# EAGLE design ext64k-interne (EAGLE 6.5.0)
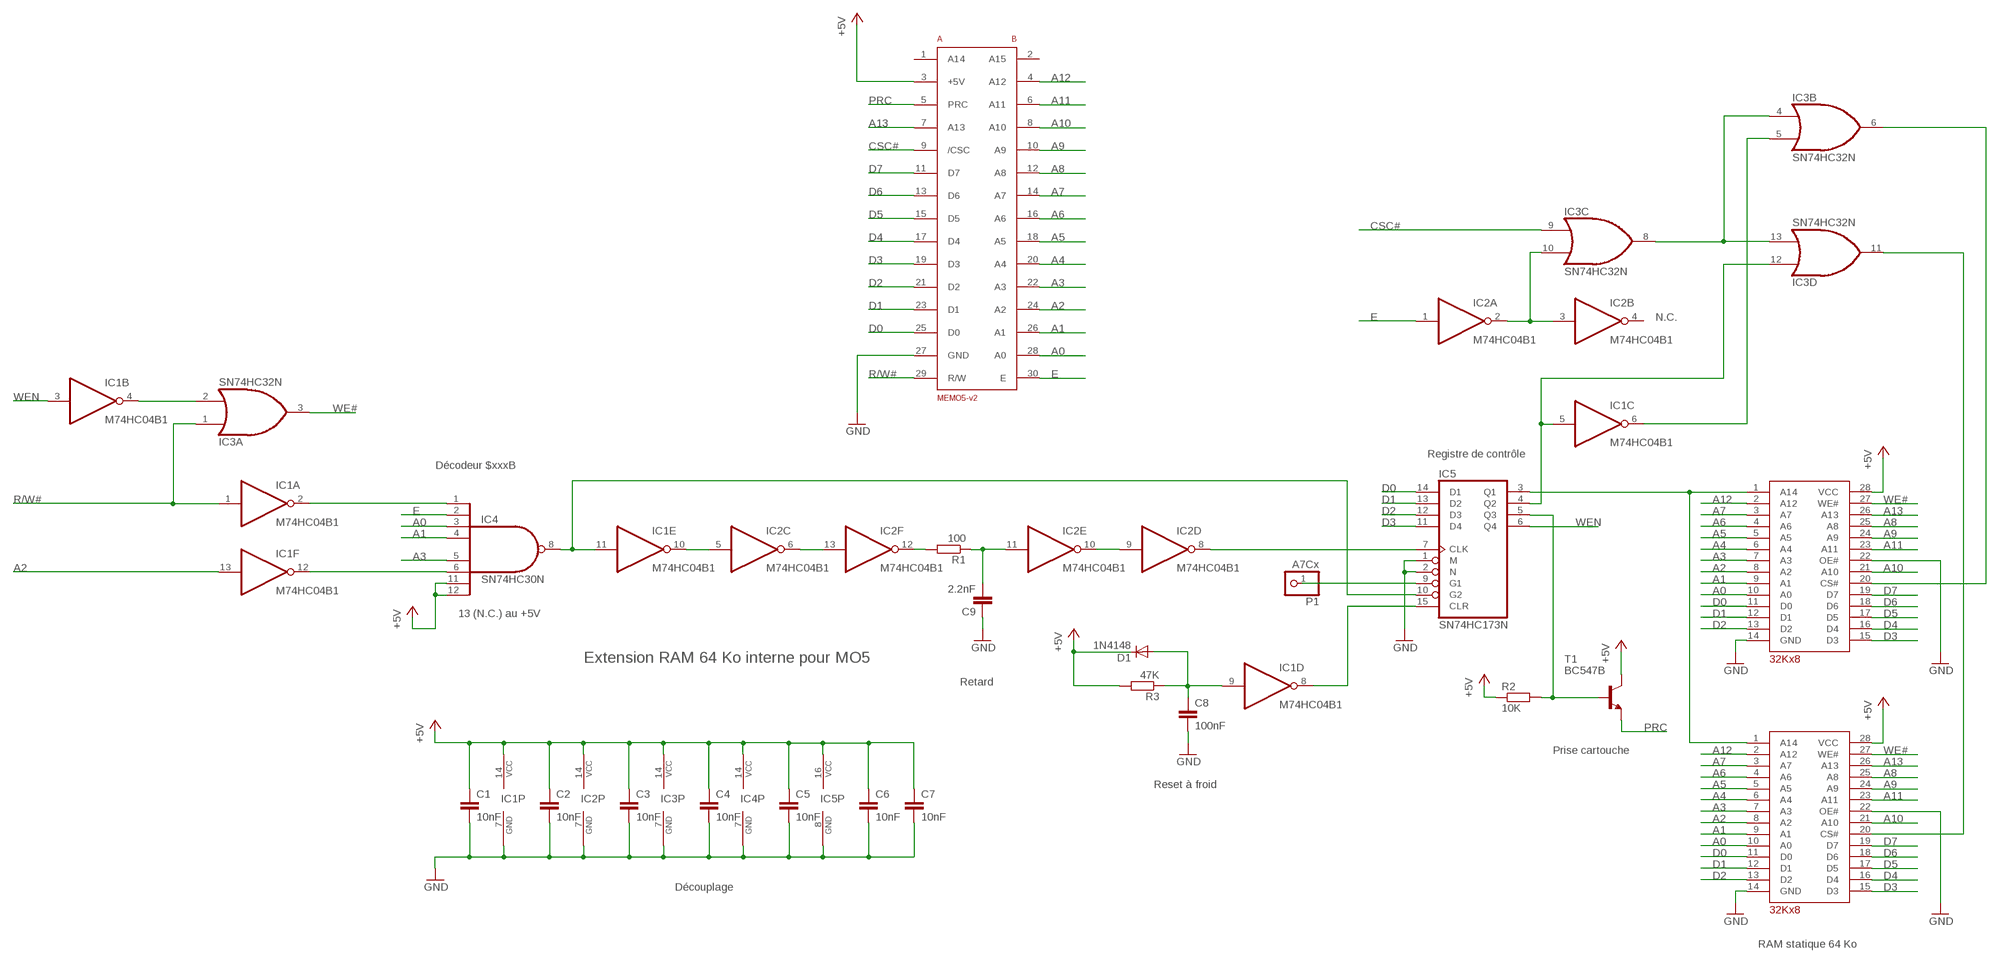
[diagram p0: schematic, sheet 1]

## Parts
C1  10nF  C-EU025-024X044  [C025-024X044]
C2  10nF  C-EU025-024X044  [C025-024X044]
C3  10nF  C-EU025-024X044  [C025-024X044]
C4  10nF  C-EU025-024X044  [C025-024X044]
C5  10nF  C-EU025-024X044  [C025-024X044]
C6  10nF  C-EU025-024X044  [C025-024X044]
C7  10nF  C-EU025-024X044  [C025-024X044]
C8  100nF  C-EU050-025X075  [C050-025X075]
C9  2.2nF  C-EU025-024X044  [C025-024X044]
D1  1N4148  1N4148DO35-10  [DO35-10]
IC1  M74HC04B1  74AS04N  [DIL14]
IC2  M74HC04B1  74AS04N  [DIL14]
IC3  SN74HC32N  74LS32N  [DIL14]
IC4  SN74HC30N  74ALS30N  [DIL14]
IC5  SN74HC173N  74LS173N  [DIL16]
IC6  D43256AC-10NL  D43256  [DIL28-6]
IC7  D43256AC-10NL  D43256  [DIL28-6]
P1  A7Cx  PINHD-1X1  [1X01]
R1  100  R-EU_0207/10  [0207/10]
R2  10K  R-EU_0207/10  [0207/10]
R3  47K  R-EU_0207/10  [0207/10]
T1  BC547B  BC547  [TO92]
U$1  MEMO5-V2HE  [HE15]

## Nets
+5V: C1.1 C2.1 C3.1 C4.1 C5.1 C6.1 C7.1 D1.C IC1.14(P:VCC) IC2.14(P:VCC) IC3.14(P:VCC) IC4.11(I6) IC4.12(I7) IC4.14(VCC) IC5.16(VCC) IC6.28(VCC) IC7.28(VCC) R2.1 R3.2 T1.3(C) U$1.3(+5V)
A0: IC4.3(I2) IC6.10(A0) IC7.10(A0) U$1.28(A0)
A1: IC4.4(I3) IC6.9(A1) IC7.9(A1) U$1.26(A1)
A2: IC1.13(F:I) IC6.8(A2) IC7.8(A2) U$1.24(A2)
A3: IC4.5(I4) IC6.7(A3) IC7.7(A3) U$1.22(A3)
A4: IC6.6(A4) IC7.6(A4) U$1.20(A4)
A5: IC6.5(A5) IC7.5(A5) U$1.18(A5)
A6: IC6.4(A6) IC7.4(A6) U$1.16(A6)
A7: IC6.3(A7) IC7.3(A7) U$1.14(A7)
A8: IC6.25(A8) IC7.25(A8) U$1.12(A8)
A9: IC6.24(A9) IC7.24(A9) U$1.10(A9)
A10: IC6.21(A10) IC7.21(A10) U$1.8(A10)
A11: IC6.23(A11) IC7.23(A11) U$1.6(A11)
A12: IC6.2(A12) IC7.2(A12) U$1.4(A12)
A13: IC6.26(A13) IC7.26(A13) U$1.7(A13)
CSC#: IC3.9(C:I0) U$1.9(/CSC)
D0: IC5.14(D1) IC6.11(D0) IC7.11(D0) U$1.25(D0)
D1: IC5.13(D2) IC6.12(D1) IC7.12(D1) U$1.23(D1)
D2: IC5.12(D3) IC6.13(D2) IC7.13(D2) U$1.21(D2)
D3: IC5.11(D4) IC6.15(D3) IC7.15(D3) U$1.19(D3)
D4: IC6.16(D4) IC7.16(D4) U$1.17(D4)
D5: IC6.17(D5) IC7.17(D5) U$1.15(D5)
D6: IC6.18(D6) IC7.18(D6) U$1.13(D6)
D7: IC6.19(D7) IC7.19(D7) U$1.11(D7)
E: IC2.1(A:I) IC4.2(I1) U$1.30(E)
GND: C1.2 C2.2 C3.2 C4.2 C5.2 C6.2 C7.2 C8.2 C9.1 IC1.7(P:GND) IC2.7(P:GND) IC3.7(P:GND) IC4.7(GND) IC5.1(M) IC5.2(N) IC5.8(GND) IC6.14(GND) IC6.22(OE#) IC7.14(GND) IC7.22(OE#) U$1.27(GND)
N$1: IC5.9(G1) P1.1
N$2: C9.2 IC2.11(E:I) R1.1
N$3: IC5.5(Q3) R2.2 T1.2(B)
N$5: IC3.4(B:I0) IC3.8(C:O) IC3.13(D:I1)
N$6: IC2.12(F:O) R1.2
N$7: IC2.6(C:O) IC2.13(F:I)
N$8: IC1.10(E:O) IC2.5(C:I)
N$9: IC1.11(E:I) IC4.8(O) IC5.10(G2)
N$10: IC2.9(D:I) IC2.10(E:O)
N$11: IC2.8(D:O) IC5.7(CLK)
N$12: IC2.2(A:O) IC2.3(B:I) IC3.10(C:I1)
N$13: IC5.3(Q1) IC6.1(A14) IC7.1(A14)
N$14: IC1.6(C:O) IC3.5(B:I1)
N$15: IC1.5(C:I) IC3.12(D:I0) IC5.4(Q2)
N$16: IC3.6(B:O) IC6.20(CS#)
N$17: IC3.11(D:O) IC7.20(CS#)
N$18: C8.1 D1.A IC1.9(D:I) R3.1
N$28: IC1.4(B:O) IC3.2(A:I1)
N$43: IC1.2(A:O) IC4.1(I0)
N$44: IC1.8(D:O) IC5.15(CLR)
N$47: IC1.12(F:O) IC4.6(I5)
PRC: T1.1(E) U$1.5(PRC)
R/W#: IC1.1(A:I) IC3.1(A:I0) U$1.29(R/W)
WE#: IC3.3(A:O) IC6.27(WE#) IC7.27(WE#)
WEN: IC1.3(B:I) IC5.6(Q4)
Unconnected: IC2.4(B:O) U$1.1(A14) U$1.2(A15)

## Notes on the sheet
- N.C.
- Registre de contrôle
- Décodeur $xxxB
- 13 (N.C.) au +5V
- Extension RAM 64 Ko interne pour MO5
- Retard
- Prise cartouche
- Reset à froid
- Découplage
- RAM statique 64 Ko

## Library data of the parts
C1-C9 = rcl:C-EU: CAPACITOR, European symbol
D1 = diode:1N4148: DIODE
IC1 IC2 = 74xx-us:74*04: Hex INVERTER
IC3 = 74xx-us:74*32: Quad 2-input OR gate
IC4 = 74xx-us:74*30: 8-input NAND gate
IC5 = 74xx-us:74*173: 4-bit D type REGISTER, 3-state
IC6 IC7 = thomson_new:D43256
P1 = pinhead:PINHD-1X1: PIN HEADER
R1-R3 = rcl:R-EU_: RESISTOR, European symbol
T1 = transistor:BC547: NPN TRANSISTOR
U$1 = thomson_new:MEMO5-V2

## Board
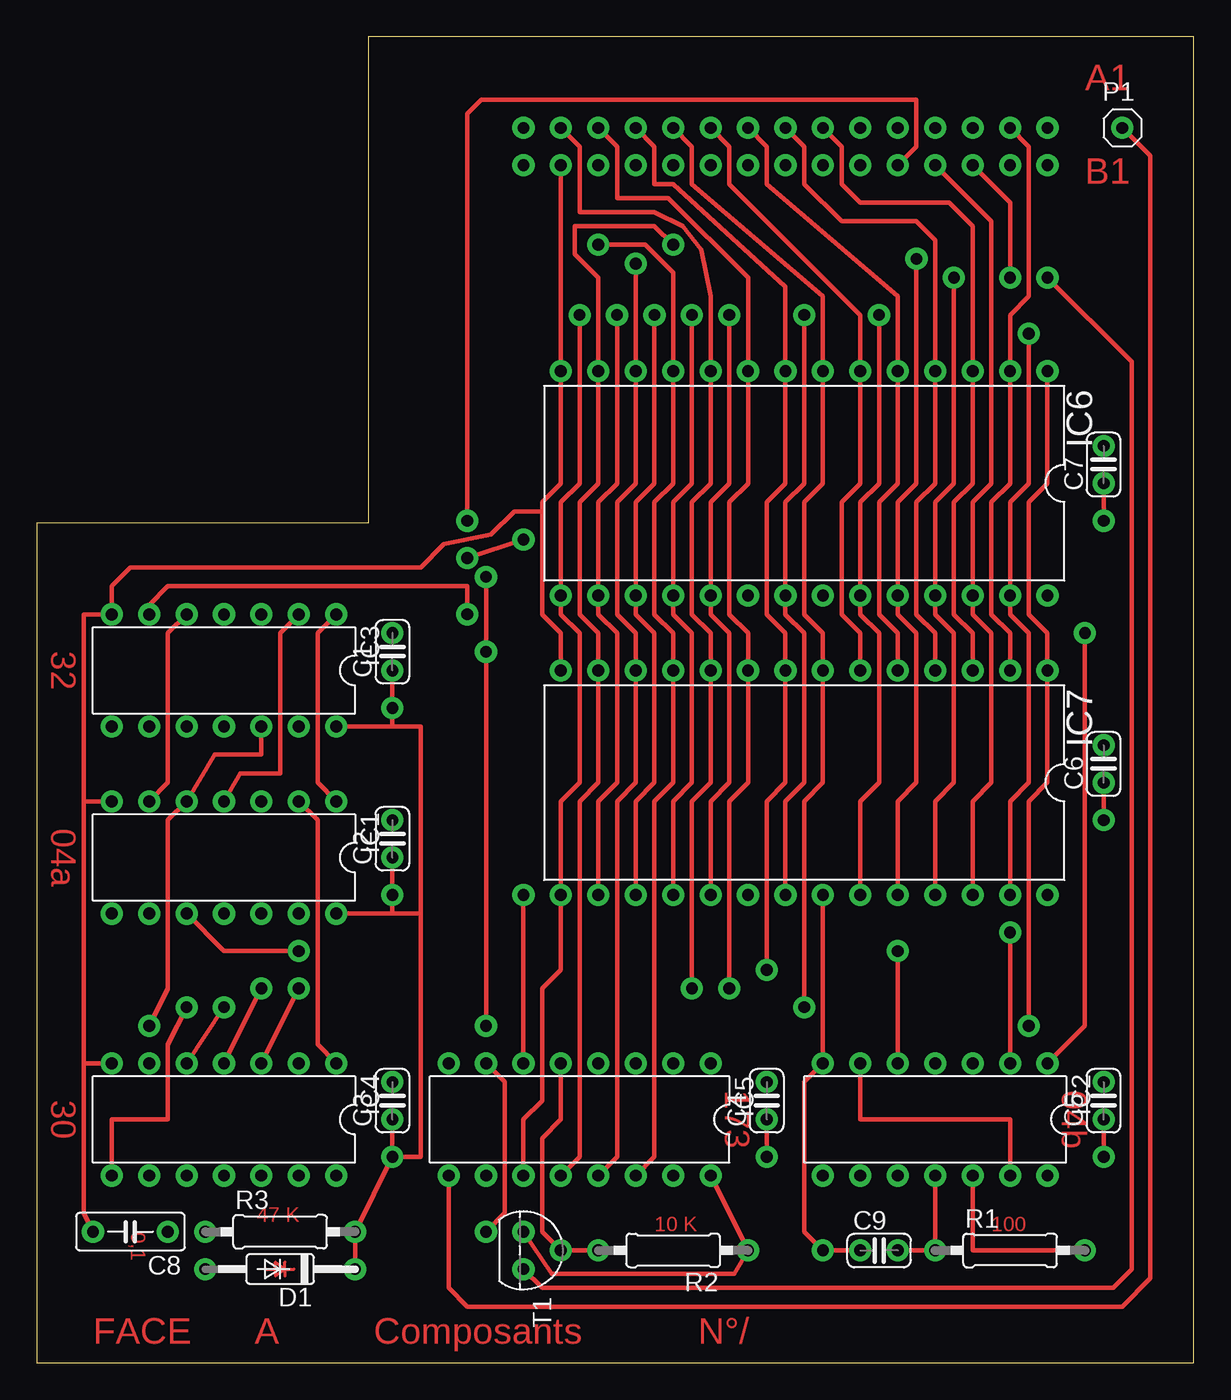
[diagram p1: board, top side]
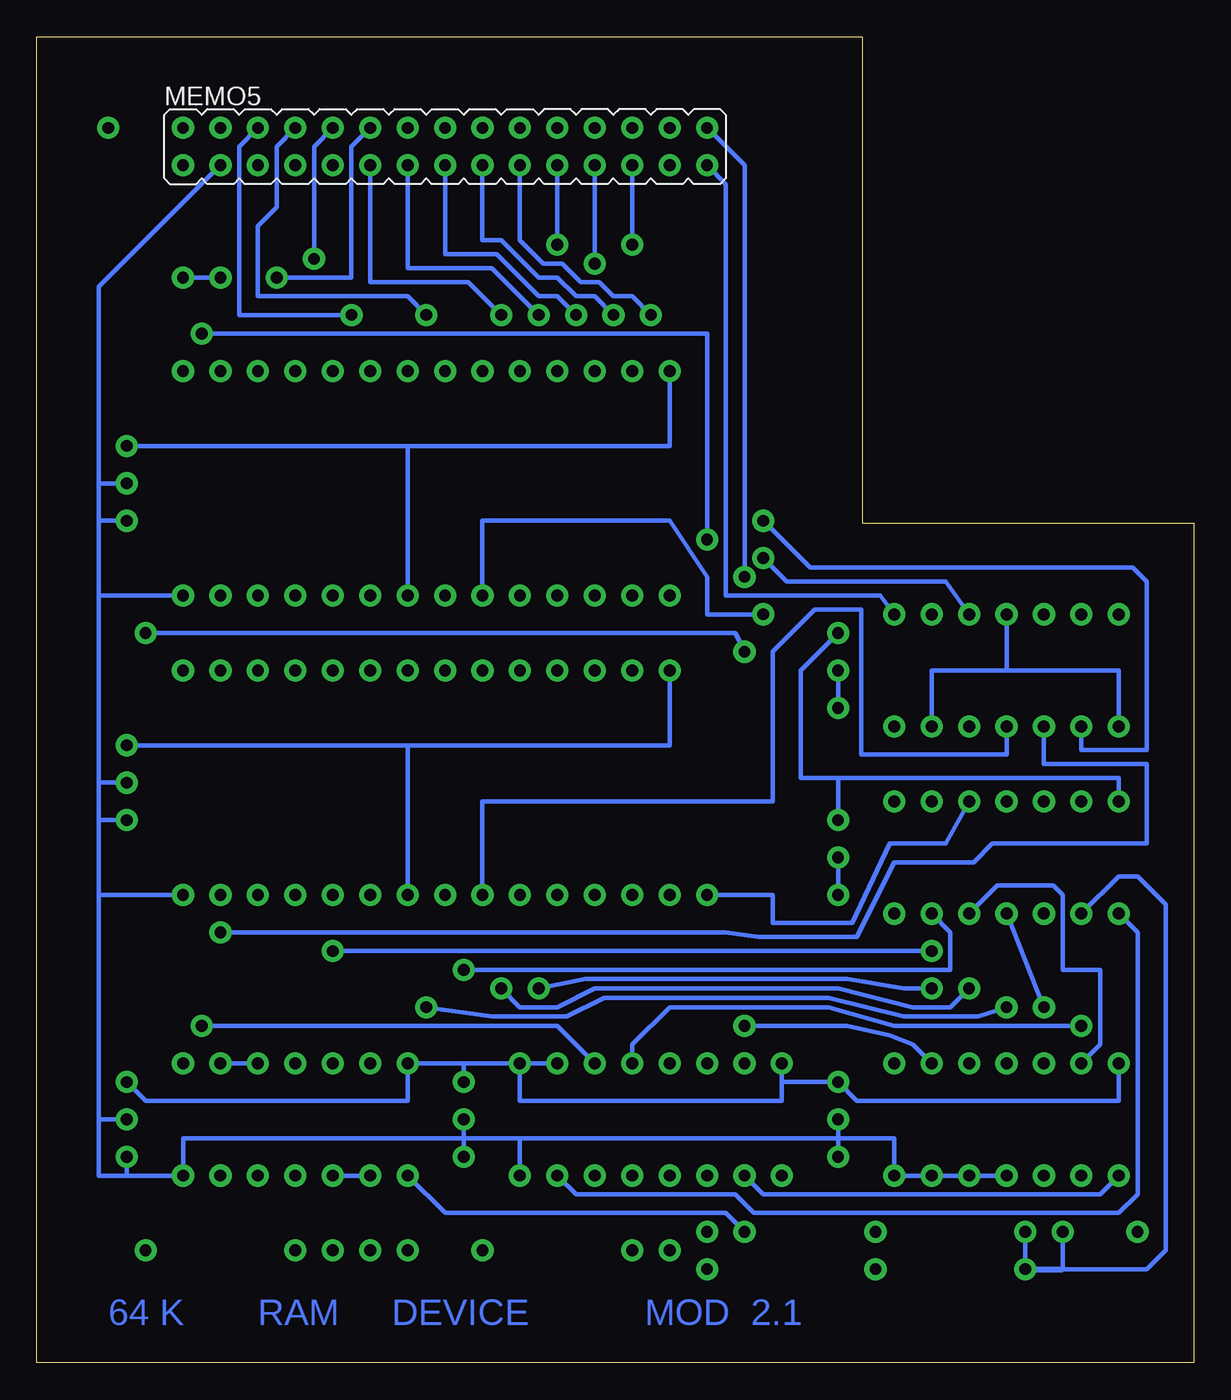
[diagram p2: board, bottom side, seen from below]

Size 78.5 x 90 mm. Coordinates in mm from the lower left corner, seen from the top.
Outline: 0,0 78.5,0 78.5,90 22.5,90 22.5,57 0,57 0,0
Copper layers (1*16): Top 0.035mm / dielectric 1.5mm / Bottom 0.035mm
Design rules "default": minimum track width 10mil, minimum drill 24mil, track to track 8mil, track to pad 8mil, pad to pad 8mil, via to via 8mil, smd to smd 8mil, copper to edge 40mil, drill to drill 8mil, minimum pad ring 10mil, minimum via ring 8mil, stop-mask expansion 4mil, vias tented up to drill 0mil, thermal gap 10mil

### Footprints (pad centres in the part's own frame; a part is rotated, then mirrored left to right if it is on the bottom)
C025-024X044 = drill 0.8 pad 1.5: 1 -1.27,0; 2 1.27,0
C050-025X075 = drill 0.8 pad 1.5: 1 -2.54,0; 2 2.54,0
DO35-10 = drill 0.8 pad 1.5: A 5.08,0; C -5.08,0
DIL14 = drill 0.813 pad 1.5: 1 -7.62,-3.81; 2 -5.08,-3.81; 3 -2.54,-3.81; 4 0,-3.81; 5 2.54,-3.81; 6 5.08,-3.81; 7 7.62,-3.81; 8 7.62,3.81; 9 5.08,3.81; 10 2.54,3.81; 11 0,3.81; 12 -2.54,3.81; 13 -5.08,3.81; 14 -7.62,3.81
DIL16 = drill 0.813 pad 1.5: 1 -8.89,-3.81; 2 -6.35,-3.81; 3 -3.81,-3.81; 4 -1.27,-3.81; 5 1.27,-3.81; 6 3.81,-3.81; 7 6.35,-3.81; 8 8.89,-3.81; 9 8.89,3.81; 10 6.35,3.81; 11 3.81,3.81; 12 1.27,3.81; 13 -1.27,3.81; 14 -3.81,3.81; 15 -6.35,3.81; 16 -8.89,3.81
DIL28-6 = drill 0.8 pad 1.5: 1 -16.51,-7.62; 2 -13.97,-7.62; 3 -11.43,-7.62; 4 -8.89,-7.62; 5 -6.35,-7.62; 6 -3.81,-7.62; 7 -1.27,-7.62; 8 1.27,-7.62; 9 3.81,-7.62; 10 6.35,-7.62; 11 8.89,-7.62; 12 11.43,-7.62; 13 13.97,-7.62; 14 16.51,-7.62; 15 16.51,7.62; 16 13.97,7.62; 17 11.43,7.62; 18 8.89,7.62; 19 6.35,7.62; 20 3.81,7.62; 21 1.27,7.62; 22 -1.27,7.62; 23 -3.81,7.62; 24 -6.35,7.62; 25 -8.89,7.62; 26 -11.43,7.62; 27 -13.97,7.62; 28 -16.51,7.62
1X01 = drill 0.8 pad 1.5: 1 0,0
0207/10 = drill 0.8 pad 1.5: 1 -5.08,0; 2 5.08,0
TO92 = drill 0.8 pad 1.5: 1 1.27,0; 2 0,2.54; 3 -1.27,0
HE15 = drill 0.8 pad 1.5: 1 -11.43,-1.27; 2 -11.43,1.27; 3 -8.89,-1.27; 4 -8.89,1.27; 5 -6.35,-1.27; 6 -6.35,1.27; 7 -3.81,-1.27; 8 -3.81,1.27; 9 -1.27,-1.27; 10 -1.27,1.27; 11 1.27,-1.27; 12 1.27,1.27; 13 3.81,-1.27; 14 3.81,1.27; 15 6.35,-1.27; 16 6.35,1.27; 17 8.89,-1.27; 18 8.89,1.27; 19 11.43,-1.27; 20 11.43,1.27; 21 13.97,-1.27; 22 13.97,1.27; 23 16.51,-1.27; 24 16.51,1.27; 25 19.05,-1.27; 26 19.05,1.27; 27 21.59,-1.27; 28 21.59,1.27; 29 24.13,-1.27; 30 24.13,1.27

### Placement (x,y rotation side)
C1  24.13,48.26 90 top
C2  24.13,35.56 90 top
C3  24.13,17.78 90 top
C4  49.53,17.78 90 top
C5  72.39,17.78 90 top
C6  72.39,40.64 90 top
C7  72.39,60.96 90 top
C8  6.35,8.89 180 top
C9  57.15,7.62 0 top
D1  16.51,6.35 180 top
IC1  12.7,34.29 180 top
IC2  60.96,16.51 180 top
IC3  12.7,46.99 180 top
IC4  12.7,16.51 180 top
IC5  36.83,16.51 180 top
IC6  52.07,59.69 180 top
IC7  52.07,39.37 180 top
P1  73.66,83.82 0 top
R1  66.04,7.62 0 top
R2  43.18,7.62 180 top
R3  16.51,8.89 0 top
T1  33.02,7.62 270 top
U$1  57.15,82.55 0 bottom

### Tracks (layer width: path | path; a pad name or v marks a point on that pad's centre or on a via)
+5V  (via drill 0.8 pad 1.5)
  Top 0.305: IC3.14 24.13,43.18 | IC1.14 24.13,30.48 | 24.13,30.48 v24.13,31.75 C2.1 | 24.13,43.18 v24.13,44.45 C1.1 | 24.13,43.18 26.04,43.18 26.04,30.48 | 26.04,30.48 24.13,30.48 | 26.04,30.48 26.04,13.97 v24.13,13.97 | C3.1 v24.13,13.97 | v24.13,13.97 R3.2 D1.C | IC5.16 R2.1 47.31,6.03 34.92,6.03 T1.3 | C4.1 v49.53,13.97 | C5.1 v72.39,13.97 | C6.1 v72.39,36.83 | v72.39,57.15 C7.1
  Bottom 0.305: IC4.11 IC4.12 IC4.14 20.32,15.24 24.13,15.24 | C3.1 24.13,15.24 | 24.13,15.24 v24.13,13.97 | 72.39,12.7 IC2.14 68.58,15.24 49.53,15.24 | 72.39,12.7 v72.39,13.97 | 72.39,12.7 74.3,12.7 74.3,16.51 | 74.3,16.51 C5.1 | 74.3,16.51 74.3,31.75 | 74.3,31.75 IC7.28 | 74.3,31.75 74.3,36.83 | 74.3,36.83 v72.39,36.83 | C6.1 74.3,39.37 | 74.3,39.37 74.3,36.83 | 74.3,39.37 74.3,52.07 | 74.3,52.07 IC6.28 | 74.3,52.07 74.3,57.15 | 74.3,57.15 v72.39,57.15 | 74.3,57.15 74.3,59.69 | 74.3,59.69 C7.1 | C4.1 49.53,15.24 | 49.53,15.24 v49.53,13.97 | 49.53,15.24 45.72,15.24 | 45.72,15.24 IC5.16 | 45.72,15.24 24.13,15.24 | 74.3,59.69 74.3,73.03 U$1.3 | v24.13,44.45 C1.1 | v24.13,31.75 C2.1
A0  (via drill 0.8 pad 1.5)
  Top 0.305: IC4.3 v17.78,25.4 | v44.45,25.4 44.45,38.1 45.72,39.37 IC7.10 45.72,49.53 44.45,50.8 44.45,58.42 45.72,59.69 IC6.10 45.72,72.39 45.09,75.56 43.81,77.15 41.91,78.11 36.83,78.11 36.83,82.55 U$1.28
  Bottom 0.305: v17.78,25.4 19.68,25.4 23.5,26.04 41.27,26.04 v44.45,25.4
A1  (via drill 0.8 pad 1.5)
  Top 0.305: IC4.4 v15.24,25.4 | v46.99,25.4 46.99,38.1 48.26,39.37 IC7.9 48.26,49.53 46.99,50.8 46.99,58.42 48.26,59.69 IC6.9 48.26,73.66 42.86,79.06 39.37,79.06 39.37,82.55 U$1.26
  Bottom 0.305: v15.24,25.4 16.51,24.13 19.05,24.13 24.13,25.4 40.64,25.4 43.18,24.13 45.72,24.13 v46.99,25.4
A2  (via drill 0.8 pad 1.5)
  Top 0.305: v49.53,26.67 49.53,38.1 50.8,39.37 IC7.8 50.8,49.53 49.53,50.8 49.53,58.42 50.8,59.69 IC6.8 50.8,73.03 43.18,80.01 41.91,80.01 41.91,82.55 U$1.24
  Bottom 0.305: IC1.13 16.51,29.21 16.51,26.67 v49.53,26.67
A3  (via drill 0.8 pad 1.5)
  Top 0.305: IC4.5 v12.7,24.13 | v52.07,24.13 52.07,38.1 53.34,39.37 IC7.7 53.34,49.53 52.07,50.8 52.07,58.42 53.34,59.69 IC6.7 53.34,72.39 44.45,80.01 44.45,82.55 U$1.22
  Bottom 0.305: v12.7,24.13 14.61,23.5 19.68,23.5 24.77,24.77 40.01,24.77 42.55,23.5 47.62,23.5 v52.07,24.13
A4
  Top 0.305: IC7.6 55.88,49.53 54.61,50.8 54.61,58.42 55.88,59.69 IC6.6 55.88,71.12 46.99,80.01 46.99,82.55 U$1.20
A5
  Top 0.305: IC7.5 58.42,49.53 57.15,50.8 57.15,58.42 58.42,59.69 IC6.5 58.42,72.39 49.53,80.01 49.53,82.55 U$1.18
A6
  Top 0.305: IC7.4 60.96,49.53 59.69,50.8 59.69,58.42 60.96,59.69 IC6.4 60.96,76.2 59.69,77.47 54.61,77.47 52.07,80.01 52.07,82.55 U$1.16
A7
  Top 0.305: IC7.3 63.5,49.53 62.23,50.8 62.23,58.42 63.5,59.69 IC6.3 63.5,77.15 61.91,78.74 55.88,78.74 54.61,80.01 54.61,82.55 U$1.14
A8  (via drill 0.8 pad 1.5)
  Top 0.305: IC7.25 60.96,38.1 62.23,39.37 62.23,49.53 60.96,50.8 IC6.25 60.96,58.42 62.23,59.69 v62.23,73.66
  Bottom 0.305: v62.23,73.66 57.15,73.66 57.15,82.55 U$1.12
A9  (via drill 0.8 pad 1.5)
  Top 0.305: IC7.24 58.42,38.1 59.69,39.37 59.69,49.53 58.42,50.8 IC6.24 58.42,58.42 59.69,59.69 v59.69,74.93
  Bottom 0.305: v59.69,74.93 59.69,82.55 U$1.10
A10  (via drill 0.8 pad 1.5)
  Top 0.305: IC7.21 50.8,38.1 52.07,39.37 52.07,49.53 50.8,50.8 IC6.21 50.8,58.42 52.07,59.69 v52.07,71.12
  Bottom 0.305: v52.07,71.12 53.34,72.39 63.5,72.39 63.5,77.15 62.23,78.42 62.23,82.55 U$1.8
A11  (via drill 0.8 pad 1.5)
  Top 0.305: IC7.23 55.88,38.1 57.15,39.37 57.15,49.53 55.88,50.8 IC6.23 55.88,58.42 57.15,59.69 v57.15,71.12
  Bottom 0.305: v57.15,71.12 64.77,71.12 64.77,82.55 U$1.6
A12
  Top 0.305: IC7.2 66.04,49.53 64.77,50.8 64.77,58.42 66.04,59.69 IC6.2 66.04,71.12 67.31,72.39 67.31,82.55 U$1.4
A13
  Top 0.305: IC7.26 63.5,38.1 64.77,39.37 64.77,49.53 63.5,50.8 IC6.26 63.5,58.42 64.77,59.69 64.77,77.47 U$1.7
CSC#  (via drill 0.8 pad 1.5)
  Top 0.305: U$1.9 59.69,82.55 59.69,85.72 30.16,85.72 29.21,84.77 v29.21,57.15
  Bottom 0.305: IC3.9 7.62,41.59 3.17,41.59 3.17,53.02 4.13,53.98 26.04,53.98 v29.21,57.15
D0  (via drill 0.8 pad 1.5)
  Top 0.305: IC5.14 41.91,13.97 41.91,38.1 43.18,39.37 IC7.11 43.18,49.53 41.91,50.8 41.91,58.42 43.18,59.69 IC6.11 43.18,73.98 41.27,75.88 v38.1,75.88
  Bottom 0.305: v38.1,75.88 U$1.25
D1  (via drill 0.8 pad 1.5)
  Top 0.305: IC5.13 39.37,13.97 39.37,38.1 40.64,39.37 IC7.12 40.64,49.53 39.37,50.8 39.37,58.42 40.64,59.69 IC6.12 v40.64,74.61
  Bottom 0.305: v40.64,74.61 U$1.23
D2  (via drill 0.8 pad 1.5)
  Top 0.305: IC5.12 36.83,13.97 36.83,38.1 38.1,39.37 IC7.13 38.1,49.53 36.83,50.8 36.83,58.42 38.1,59.69 IC6.13 38.1,73.66 36.51,75.25 36.51,77.15 41.91,77.15 v43.18,75.88
  Bottom 0.305: v43.18,75.88 U$1.21
D3  (via drill 0.8 pad 1.5)
  Top 0.305: IC5.11 33.02,16.51 34.29,17.78 34.29,25.4 35.56,26.67 IC7.15 35.56,38.1 36.83,39.37 36.83,49.53 35.56,50.8 IC6.15 35.56,58.42 36.83,59.69 v36.83,71.12
  Bottom 0.305: v36.83,71.12 38.1,72.39 39.37,72.39 40.32,73.34 41.59,73.34 42.86,74.61 44.13,74.61 45.72,76.2 U$1.19
D4  (via drill 0.8 pad 1.5)
  Top 0.305: IC7.16 38.1,38.1 39.37,39.37 39.37,49.53 38.1,50.8 IC6.16 38.1,58.42 39.37,59.69 v39.37,71.12
  Bottom 0.305: v39.37,71.12 40.64,72.39 41.91,72.39 43.18,73.66 44.45,73.66 46.99,76.2 48.26,76.2 48.26,77.47 U$1.17
D5  (via drill 0.8 pad 1.5)
  Top 0.305: IC7.17 40.64,38.1 41.91,39.37 41.91,49.53 40.64,50.8 IC6.17 40.64,58.42 41.91,59.69 v41.91,71.12
  Bottom 0.305: v41.91,71.12 43.18,72.39 44.45,72.39 47.31,75.25 50.8,75.25 U$1.15
D6  (via drill 0.8 pad 1.5)
  Top 0.305: IC7.18 43.18,38.1 44.45,39.37 44.45,49.53 43.18,50.8 IC6.18 43.18,58.42 44.45,59.69 v44.45,71.12
  Bottom 0.305: v44.45,71.12 47.62,74.3 53.34,74.3 U$1.13
D7  (via drill 0.8 pad 1.5)
  Top 0.305: v46.99,71.12 46.99,59.69 45.72,58.42 IC6.19 45.72,50.8 46.99,49.53 46.99,39.37 45.72,38.1 IC7.19
  Bottom 0.305: v46.99,71.12 49.21,73.34 55.88,73.34 U$1.11
E  (via drill 0.8 pad 1.5)
  Top 0.305: IC2.1 71.12,22.86 v71.12,49.53 | v30.48,22.86 v30.48,48.26 v30.48,53.34
  Bottom 0.305: v71.12,49.53 31.11,49.53 v30.48,48.26 | v30.48,22.86 23.5,22.86 20.64,22.23 19.05,21.59 IC4.2 | v30.48,53.34 30.48,81.28 U$1.30
GND  (via drill 0.8 pad 1.5)
  Top 0.305: 3.17,38.1 3.17,50.8 IC3.7 5.08,52.7 6.35,53.98 26.04,53.98 27.62,55.56 30.8,56.2 32.38,57.78 34.29,57.78 | 3.17,38.1 IC1.7 | 3.17,38.1 3.17,20.32 | 3.17,20.32 IC4.7 | 3.17,20.32 3.17,10.16 C8.2 | IC7.14 35.56,49.53 34.29,50.8 34.29,57.78 | 34.29,57.78 34.29,58.42 35.56,59.69 IC6.14 U$1.27 | IC7.22 IC2.7 52.07,19.05 52.07,8.89 v53.34,7.62 C9.1
  Bottom 0.305: 27.94,19.05 C3.2 22.86,17.78 5.08,17.78 IC4.7 | 27.94,19.05 IC5.8 | C7.2 53.34,62.23 | 53.34,62.23 IC6.22 | C6.2 53.34,41.91 | 53.34,41.91 IC7.22 | 53.34,41.91 35.56,41.91 IC7.14 | 53.34,62.23 35.56,62.23 IC6.14 | C5.2 71.12,17.78 53.34,17.78 IC2.7 49.53,20.32 | 49.53,20.32 IC5.1 | 49.53,20.32 C4.2 | IC5.1 IC5.2 | IC5.1 45.72,17.78 27.94,17.78 27.94,19.05 | IC1.7 5.08,39.69 24.13,39.69 | 24.13,39.69 C2.2 | 24.13,39.69 26.67,39.69 26.67,46.99 C1.2
N$1
  Top 0.305: IC5.9 27.94,5.08 29.21,3.81 73.66,3.81 75.56,5.71 75.56,81.92 P1.1
N$2
  Top 0.305: IC2.11 R1.1 C9.2
N$3
  Top 0.305: IC5.5 35.56,16.51 34.29,15.24 34.29,8.89 T1.2 R2.2
N$4
  Top 0.2: 15.56,6.35 16.19,6.35 | 16.19,6.35 16.19,6.83 16.83,6.35 | 16.19,6.35 16.19,5.87 16.83,6.35 | 16.83,6.35 16.83,6.83 | 16.83,6.35 16.83,5.87 | 16.83,6.35 17.46,6.35
N$5
  Bottom 0.305: IC3.4 12.7,46.99 | 12.7,46.99 17.78,46.99 IC3.13 | 12.7,46.99 5.08,46.99 IC3.8
N$6
  Top 0.305: IC2.12 63.5,7.62 R1.2
N$7
  Top 0.305: IC2.13 66.04,16.51 55.88,16.51 IC2.6
N$8  (via drill 0.8 pad 1.5)
  Top 0.305: IC1.10 12.7,27.94 v17.78,27.94 | IC2.5 v58.42,27.94
  Bottom 0.305: v17.78,27.94 v58.42,27.94
N$9  (via drill 0.8 pad 1.5)
  Top 0.305: IC4.8 5.08,16.51 8.89,16.51 8.89,21.59 v10.16,24.13
  Bottom 0.305: v10.16,24.13 IC1.11 | IC5.10 29.21,11.43 6.35,11.43 IC4.8
N$10
  Bottom 0.305: IC2.9 IC2.10
N$11  (via drill 0.8 pad 1.5)
  Top 0.305: IC5.7 31.75,19.05 31.75,10.16 v30.48,8.89
  Bottom 0.305: IC2.8 50.8,10.16 31.75,10.16 v30.48,8.89
N$12  (via drill 0.8 pad 1.5)
  Top 0.305: IC2.2 v66.04,29.21
  Bottom 0.305: IC2.3 IC2.2 | v66.04,29.21 31.75,29.21 29.53,28.89 22.86,28.89 20.32,33.97 14.92,33.97 13.65,35.24 3.17,35.24 3.17,40.64 10.16,40.64 IC3.10
N$13  (via drill 0.8 pad 1.5)
  Top 0.305: IC6.1 68.58,59.69 67.31,58.42 67.31,50.8 68.58,49.53 IC7.1 68.58,39.37 67.31,38.1 v67.31,22.86
  Bottom 0.305: v67.31,22.86 43.18,22.86 IC5.3
N$14
  Top 0.305: IC3.5 8.89,49.53 8.89,39.37 IC1.6
N$15  (via drill 0.8 pad 1.5)
  Top 0.305: IC3.12 15.24,41.27 12.06,41.27 IC1.5 8.89,36.83 8.89,25.4 v7.62,22.86
  Bottom 0.305: IC5.4 38.1,21.59 35.56,24.13 24.77,24.13 20.32,22.86 v7.62,22.86
N$16  (via drill 0.8 pad 1.5)
  Top 0.305: IC3.6 7.62,51.44 8.89,52.7 29.21,52.7 v29.21,50.8
  Bottom 0.305: v29.21,50.8 33.02,50.8 33.02,53.34 35.56,57.15 48.26,57.15 IC6.20
N$17
  Bottom 0.305: IC3.11 12.7,41.27 22.54,41.27 22.54,51.12 25.72,51.12 28.57,48.26 28.57,38.1 48.26,38.1 IC7.20
N$18
  Bottom 0.305: D1.A R3.1 | C8.1 8.89,6.35 3.17,6.35 1.91,7.62 1.91,31.11 3.81,33.02 5.08,33.02 IC1.9
  Bottom 0.406: D1.A 8.89,6.35
N$28
  Top 0.305: IC3.2 16.51,49.53 16.51,40.01 13.81,40.01 IC1.4
N$43
  Top 0.305: IC4.1 19.05,21.59 19.05,36.83 IC1.2
N$44
  Bottom 0.305: IC5.15 41.91,11.43 31.11,11.43 29.84,10.16 5.08,10.16 3.81,11.43 3.81,29.21 IC1.8
N$47
  Bottom 0.305: IC4.6 6.35,21.59 6.35,26.67 8.89,26.67 8.89,31.75 9.53,32.38 13.34,32.38 IC1.12
PRC  (via drill 0.8 pad 1.5)
  Top 0.305: T1.1 34.29,5.08 73.03,5.08 74.3,6.35 74.3,67.94 v68.58,73.66 | U$1.5 66.04,78.74 v66.04,73.66
  Bottom 0.305: v66.04,73.66 v68.58,73.66
R/W#
  Top 0.305: IC1.1 19.05,39.37 19.05,49.53 IC3.1
  Bottom 0.305: IC3.1 21.27,52.07 31.75,52.07 31.75,80.01 U$1.29
WE#  (via drill 0.8 pad 1.5)
  Top 0.305: IC7.27 66.04,38.1 67.31,39.37 67.31,49.53 66.04,50.8 IC6.27 66.04,58.42 67.31,59.69 v67.31,69.85 | v29.21,54.61 v33.02,55.88
  Bottom 0.305: v67.31,69.85 33.02,69.85 v33.02,55.88 | IC3.3 16.83,53.02 27.62,53.02 v29.21,54.61
WEN  (via drill 0.8 pad 1.5)
  Top 0.305: IC5.6 v33.02,31.75
  Bottom 0.305: v33.02,31.75 28.57,31.75 28.57,29.84 23.18,29.84 20.64,35.24 16.83,35.24 IC1.3

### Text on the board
Top: A1 | B1 | 32 | 04a | 30 | 173 | 04b | 47 K | 0,1 | 10 K | 100 | FACE A Composants N°/
Bottom: 64 K RAM DEVICE MOD 2.1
